ORGANIZATION_BLOCK "Hardware Interrupt 2"
TITLE =
VERSION : 0.1


VAR_TEMP
  OB42_EV_CLASS : BYTE ;	//Bits 0-3 = 1 (Coming event), Bits 4-7 = 1 (Event class 1)
  OB42_STRT_INF : BYTE ;	//16#41/42/43/44 (Interrupt 1/2/3/4)
  OB42_PRIORITY : BYTE ;	//18 (Priority of 1 is lowest)
  OB42_OB_NUMBR : BYTE ;	//42 (Organization block 42, OB42)
  OB42_RESERVED_1 : BYTE ;	//Reserved for system
  OB42_RESERVED_2 : BYTE ;	//Reserved for system
  OB42_MDL_ADDR : WORD ;	//Base address of module initiating interrupt
  OB42_POINT_ADDR : DWORD ;	//Address of interrupt point on module
  OB42_DATE_TIME : DATE_AND_TIME ;	//Date and time OB42 started
END_VAR
BEGIN
END_ORGANIZATION_BLOCK

